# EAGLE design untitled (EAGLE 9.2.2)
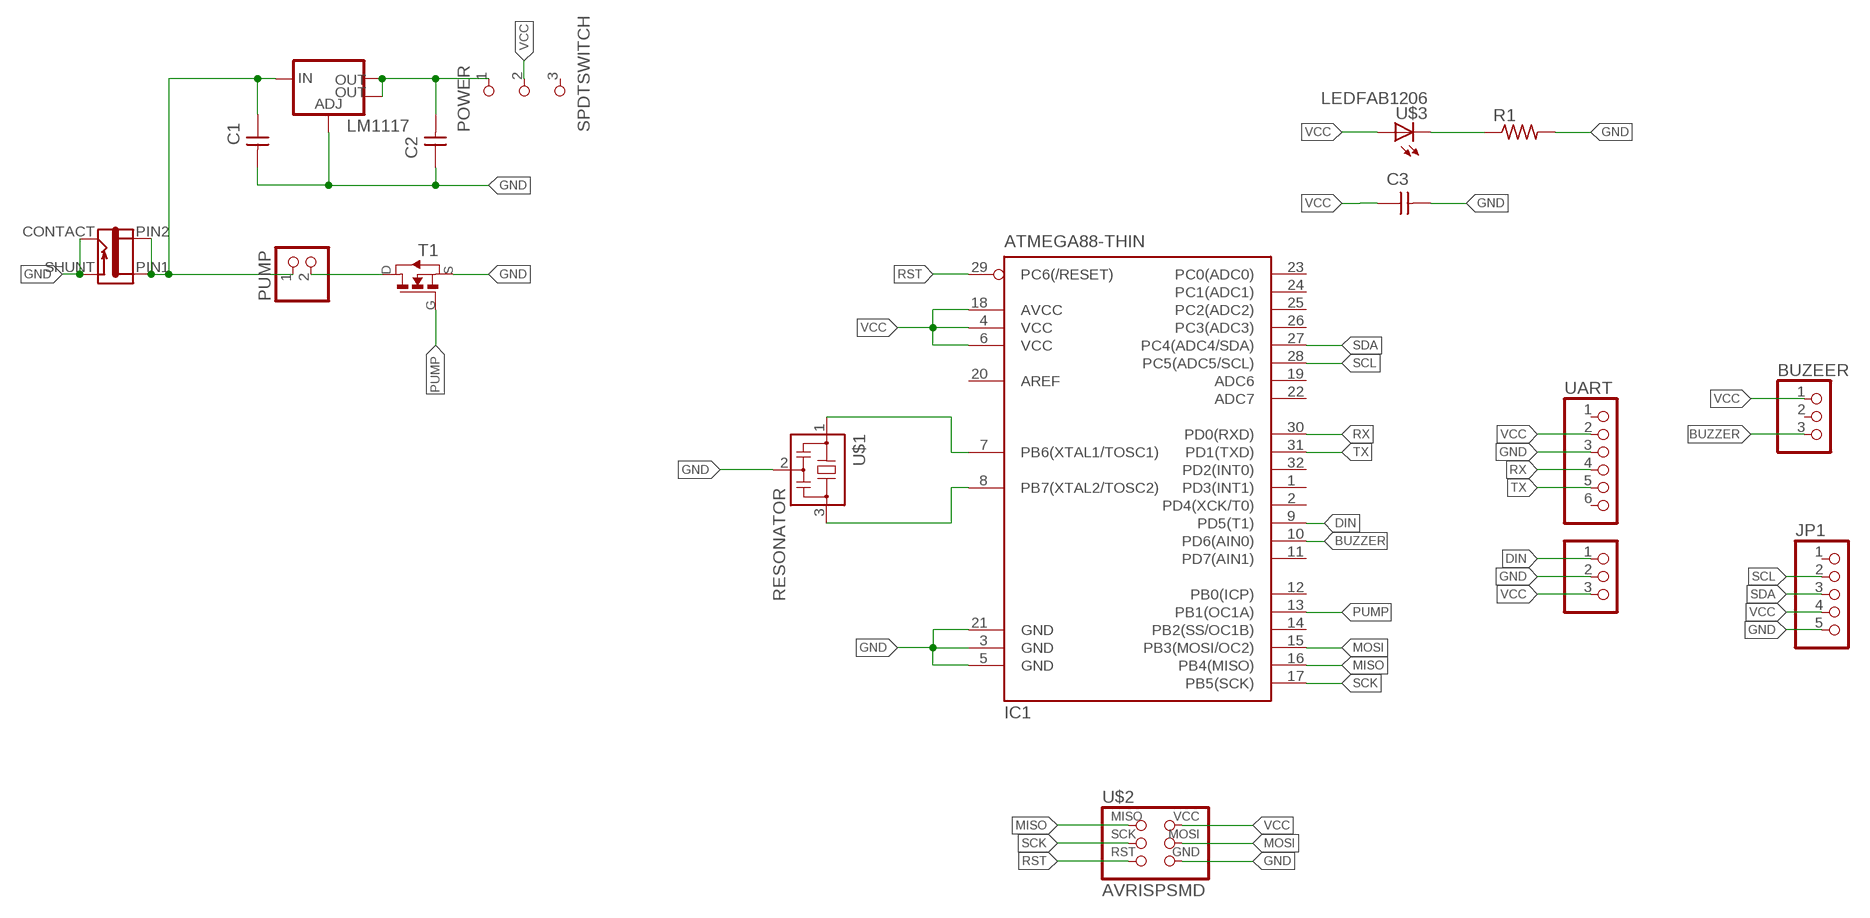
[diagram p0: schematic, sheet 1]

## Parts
BUZEER  PINHD-1X3/90  [1X03/90]
C1  CAP-UNPOLARIZEDFAB  [C1206FAB]
C2  CAP-UNPOLARIZEDFAB  [C1206FAB]
C3  CAP-UNPOLARIZEDFAB  [C1206FAB]
IC1  ATMEGA88-THIN  [TQFP32-08THIN]
J1  JACK-2.1MM  [PJ-002AH-SMT]
JP1  PINHD-1X5/90  [1X05/90]
LM1117  V_REG_LM1117SOT223  [SOT223]
NEO  PINHD-1X3/90  [1X03/90]
POWER  SPDTSWITCH  [SPDTSWITCH]
PUMP  PINHD-1X2  [1X02]
R1  RES-US1206FAB  [R1206FAB]
T1  NMOSFETTO252  [TO252]
U$1  RESONATOR  [EFOBM]
U$2  AVRISPSMD  [2X03SMD]
U$3  LEDFAB1206  [LED1206FAB]
UART  PINHD-1X6/90  [1X06/90]

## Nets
BUZZER: BUZEER.3 IC1.10(PD6(AIN0))
DIN: IC1.9(PD5(T1)) NEO.1
GND: C1.2 C2.1 C3.2 IC1.3(GND) IC1.5(GND) IC1.21(GND) J1.CONTACT J1.SHUNT JP1.5 LM1117.1(ADJ) NEO.2 R1.2 T1.2(S) U$1.2 U$2.6(GND) UART.3
MISO: IC1.16(PB4(MISO)) U$2.1(MISO)
MOSI: IC1.15(PB3(MOSI/OC2)) U$2.4(MOSI)
N$1: C2.2 LM1117.2(OUT) LM1117.4(OUT) POWER.1
N$2: PUMP.2 T1.3(D)
N$3: C1.1 J1.PIN1 J1.PIN2 LM1117.3(IN) PUMP.1
N$4: R1.1 U$3.2(C)
N$5: IC1.7(PB6(XTAL1/TOSC1)) U$1.1
N$6: IC1.8(PB7(XTAL2/TOSC2)) U$1.3
PUMP: IC1.13(PB1(OC1A)) T1.1(G)
RST: IC1.29(PC6(/RESET)) U$2.5(RST)
RX: IC1.30(PD0(RXD)) UART.4
SCK: IC1.17(PB5(SCK)) U$2.3(SCK)
SCL: IC1.28(PC5(ADC5/SCL)) JP1.2
SDA: IC1.27(PC4(ADC4/SDA)) JP1.3
TX: IC1.31(PD1(TXD)) UART.5
VCC: BUZEER.1 C3.1 IC1.4(VCC) IC1.6(VCC) IC1.18(AVCC) JP1.4 NEO.3 POWER.2 U$2.2(VCC) U$3.1(A) UART.2
Unconnected: BUZEER.2 IC1.1(PD3(INT1)) IC1.2(PD4(XCK/T0)) IC1.11(PD7(AIN1)) IC1.12(PB0(ICP)) IC1.14(PB2(SS/OC1B)) IC1.19(ADC6) IC1.20(AREF) IC1.22(ADC7) IC1.23(PC0(ADC0)) IC1.24(PC1(ADC1)) IC1.25(PC2(ADC2)) IC1.26(PC3(ADC3)) IC1.32(PD2(INT0)) JP1.1 POWER.3 UART.1 UART.6

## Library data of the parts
BUZEER NEO = pinhead:PINHD-1X3: PIN HEADER
C1-C3 = fab:CAP-UNPOLARIZED
IC1 = fab:ATMEGA88-THIN
J1 = fab:JACK-2.1MM: SMD DC power jack PJ-002AH-SMT As found in the fablab inventory. Made by Zaerc.
JP1 = pinhead:PINHD-1X5: PIN HEADER
LM1117 = fab:V_REG_LM1117: Voltage Regulator LM1117 Standard adjustable voltage regulator but in SMD form. Spark Fun Electronics SKU : COM-00595; PROD_ID: VREG-08170
POWER = fab:SPDTSWITCH
PUMP = pinhead:PINHD-1X2: PIN HEADER
R1 = fab:RES-US: Resistor (US Symbol)
T1 = fab:NMOSFET: MOS FET
U$1 = fab:RESONATOR
U$2 = fab:AVRISP
U$3 = fab:LED: LED
UART = pinhead:PINHD-1X6: PIN HEADER

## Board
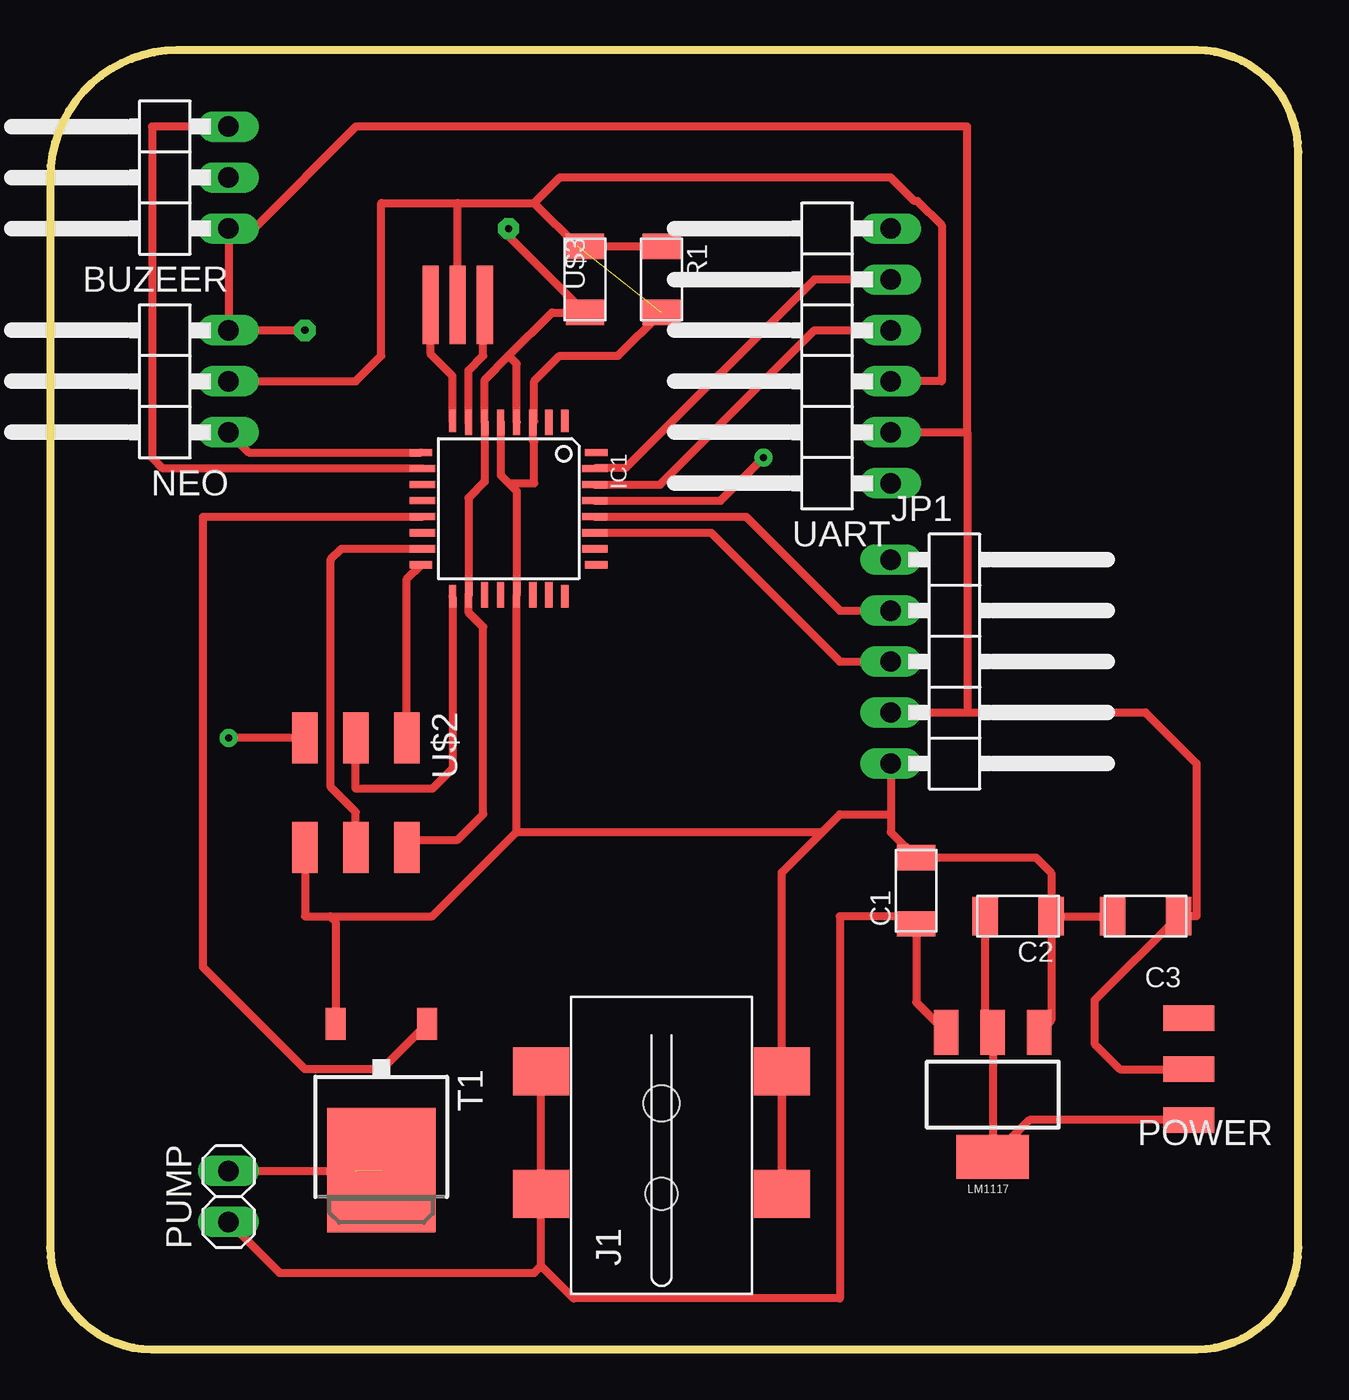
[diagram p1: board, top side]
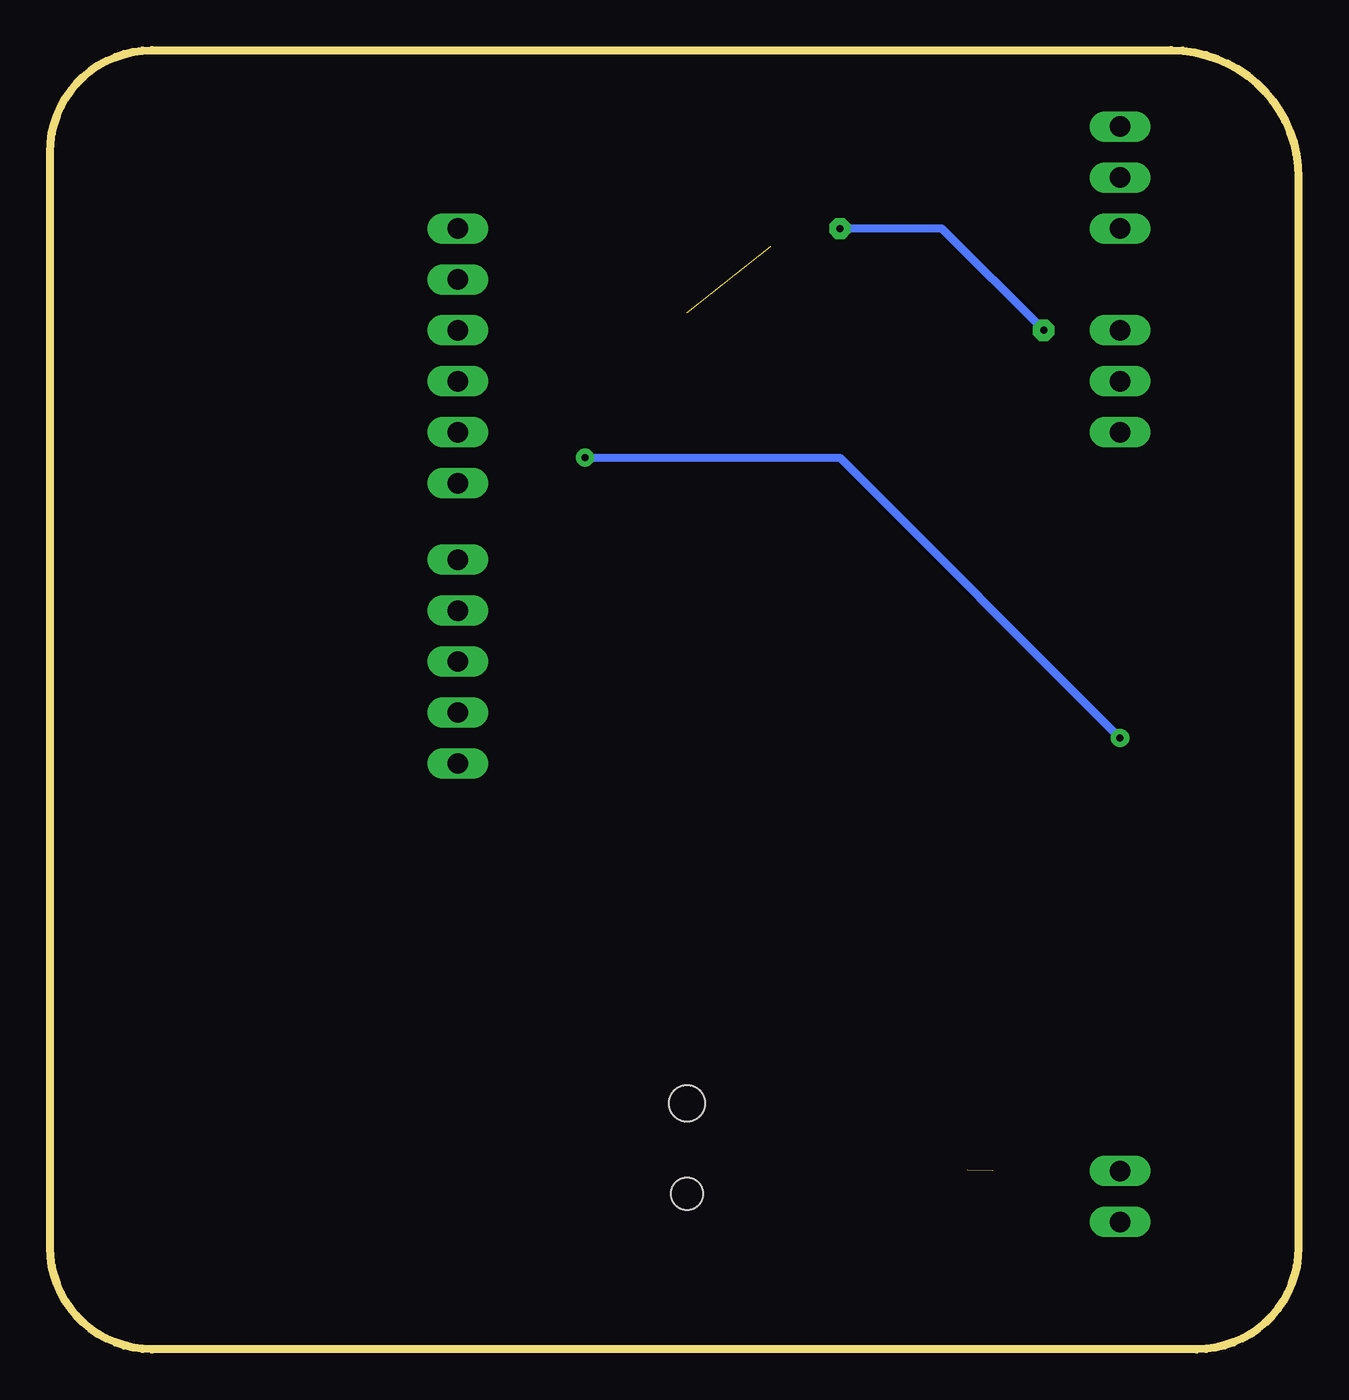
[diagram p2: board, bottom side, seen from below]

Size 62.23 x 64.77 mm. Coordinates in mm from the lower left corner, seen from the top.
Outline: 6.35,64.77 arc90 0,58.42 0,5.08 arc90 5.08,0 57.15,0 arc90 62.23,5.08 62.23,59.69 arc90 57.15,64.77 6.35,64.77
Copper layers (1*16): Top 0.035mm / dielectric 1.5mm / Bottom 0.035mm
Design rules "default *": minimum track width 16mil, minimum drill 0.35mm, track to track 16mil, track to pad 16mil, pad to pad 16mil, via to via 16mil, smd to smd 16mil, copper to edge 16mil, drill to drill 16mil, minimum pad ring 10mil, minimum via ring 8mil, stop-mask expansion 4mil, vias tented up to drill 0mil, thermal gap 10mil

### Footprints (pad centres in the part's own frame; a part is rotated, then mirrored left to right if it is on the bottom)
1X03/90 = drill 1.016 long: 1 -2.54,-3.81; 2 0,-3.81; 3 2.54,-3.81
C1206FAB = smd 1.27 x 1.905: 1 -1.651,0; 2 1.651,0
TQFP32-08THIN = smd 1.118 x 0.356: 1 -4.369,2.8; 8 -4.369,-2.8; 17 4.369,-2.8; 24 4.369,2.8 | smd 1.27 x 0.356: 2 -4.293,2; 3 -4.293,1.2; 4 -4.293,0.4; 5 -4.293,-0.4; 6 -4.293,-1.2; 7 -4.293,-2; 18 4.293,-2; 19 4.293,-1.2; 20 4.293,-0.4; 21 4.293,0.4; 22 4.293,1.2; 23 4.293,2 | smd 0.356 x 1.118: 9 -2.8,-4.369; 16 2.8,-4.369; 25 2.8,4.369; 32 -2.8,4.369 | smd 0.356 x 1.27: 10 -2,-4.293; 14 1.2,-4.293; 15 2,-4.293; 26 2,4.293; 27 1.2,4.293; 31 -2,4.293 | smd 0.35 x 1.27: 11 -1.2,-4.293; 12 -0.4,-4.293; 13 0.4,-4.293; 28 0.4,4.293; 29 -0.4,4.293; 30 -1.2,4.293
PJ-002AH-SMT = smd 2.4 x 2.8: CONTACT -2.4,-6; PIN1 3.7,6; PIN2 -2.4,6; SHUNT 3.7,-6 | hole 1.6: -2.4,0 | hole 1.8: 2.1,0
1X05/90 = drill 1.016 long: 1 -5.08,-3.81; 2 -2.54,-3.81; 3 0,-3.81; 4 2.54,-3.81; 5 5.08,-3.81
SOT223 = smd 1.219 x 2.235: 1 -2.311,-3.099; 2 0,-3.099; 3 2.311,-3.099 | smd 3.6 x 2.2: 4 0,3.099
SPDTSWITCH = smd 2.54 x 1.27: 1 0.38,2.54; 2 0.38,0; 3 0.38,-2.54
1X02 = drill 1.016 long: 1 -1.27,0; 2 1.27,0
R1206FAB = smd 1.27 x 1.905: 1 -1.651,0; 2 1.651,0
TO252 = smd 1 x 1.6: 1 -2.28,-4.8; 2 2.28,-4.8 | smd 5.4 x 6.2: 3 0,2.5
EFOBM = smd 0.8 x 3.9: 1 -1.35,0; 2 0,0; 3 1.35,0
2X03SMD = smd 2.54 x 1.27: 1 -2.54,2.54; 2 2.92,2.54; 3 -2.54,0; 4 2.92,0; 5 -2.54,-2.54; 6 2.92,-2.54
LED1206FAB = smd 1.27 x 1.905: 1 -1.651,0; 2 1.651,0
1X06/90 = drill 1.016 long: 1 -6.35,-3.81; 2 -3.81,-3.81; 3 -1.27,-3.81; 4 1.27,-3.81; 5 3.81,-3.81; 6 6.35,-3.81

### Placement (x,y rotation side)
BUZEER  5.08,58.42 90 top
C1  43.18,22.86 90 top
C2  48.26,21.59 180 top
C3  54.61,21.59 180 top
IC1  22.86,41.91 270 top
J1  30.48,10.16 90 top
JP1  45.72,34.29 270 top
LM1117  46.99,12.7 180 top
NEO  5.08,48.26 90 top
POWER  57.15,13.97 180 top
PUMP  8.89,7.62 90 top
R1  30.48,53.34 270 top
T1  16.51,11.43 180 top
U$1  20.32,52.07 180 top
U$2  15.24,27.94 270 top
U$3  26.67,53.34 90 top
UART  38.1,49.53 90 top

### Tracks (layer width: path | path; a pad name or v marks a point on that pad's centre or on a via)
BUZZER
  Top 0.406: BUZEER.3 5.08,60.96 5.08,44.45 5.62,43.91 IC1.10
DIN
  Top 0.406: NEO.1 9.9,44.71 IC1.9
GND  (1 unrouted)
  Top 0.406: U$1.2 20.32,57.15 | 20.32,57.15 24.13,57.15 | 24.13,57.15 26.29,54.99 | IC1.5 22.46,43.58 22.86,43.18 | 22.86,43.18 24.13,43.18 24.13,45.26 24.07,45.31 24.07,46.19 IC1.3 24.13,46.27 24.13,48.26 25.4,49.53 28.32,49.53 R1.2 | 24.13,57.15 25.4,58.42 41.91,58.42 43.08,57.25 43.24,57.25 44.45,56.04 44.45,48.26 UART.3 | 22.86,43.18 23.26,42.78 IC1.21 23.26,25.8 | U$2.6 12.7,21.59 13.97,21.59 | 13.97,21.59 19.05,21.59 23.26,25.8 | 13.97,21.59 14.23,21.33 T1.2 | NEO.2 15.24,48.26 16.51,49.53 16.51,57.15 20.32,57.15 | C2.1 49.91,16.41 LM1117.1 | C2.1 C3.2 | C2.1 49.91,23.75 49.15,24.51 C1.2 41.91,25.78 41.91,26.67 | JP1.5 41.91,26.67 | J1.SHUNT 36.48,8.54 35.7,7.76 | 35.56,7.62 35.7,7.76 | 35.7,7.76 J1.CONTACT 36.48,23.78 38.5,25.8 | 41.91,26.67 39.37,26.67 38.5,25.8 | 23.26,25.8 38.5,25.8
MISO
  Top 0.406: U$2.1 17.78,38.4 IC1.16
MOSI
  Top 0.406: U$2.4 15.24,26.79 13.99,28.04 13.99,39.34 13.97,39.37 14.51,39.91 IC1.15
N$1
  Top 0.406: C2.2 46.61,15.62 46.99,15.24 LM1117.2 LM1117.4 48.82,11.43 POWER.1
N$2  (1 unrouted)
  Top 0.406: PUMP.2 15.24,8.89
N$3
  Top 0.406: PUMP.1 11.43,3.81 24.13,3.81 24.48,4.16 | LM1117.3 43.18,17.3 C1.1 42.8,21.59 39.37,21.59 39.37,2.54 26.1,2.54 24.48,4.16 | 24.48,4.16 J1.PIN2 J1.PIN1
N$4
  Top 0.406: U$3.2 R1.1
N$5
  Top 0.406: U$1.1 21.59,51.99 21.59,49.53 20.86,48.8 IC1.7
N$6
  Top 0.406: 19.05,51.99 U$1.3 18.97,49.61 20.06,48.52 IC1.8
PUMP
  Top 0.406: IC1.13 7.62,41.51 7.62,19.05 12.7,13.97 16.53,13.97 T1.1
RST  (via drill 0.35 pad 0.9)
  Top 0.406: IC1.29 33.42,42.31 v35.56,44.45 | U$2.5 v8.89,30.48
  Bottom 0.406: v8.89,30.48 22.86,44.45 v35.56,44.45
RX
  Top 0.406: IC1.30 30.41,43.11 38.1,50.8 UART.4
SCK
  Top 0.406: IC1.17 20.06,28.95 19.05,27.94 15.24,27.94 U$2.3
SCL
  Top 0.406: IC1.28 34.69,41.51 39.37,36.83 JP1.2
SDA
  Top 0.406: IC1.27 32.95,40.71 39.37,34.29 JP1.3
TX
  Top 0.406: UART.5 38.1,53.34 28.68,43.92 27.16,43.92 IC1.31
VCC  (via drill 0.35 pad 1.05)
  Top 0.406: 22.86,49.53 21.66,48.33 IC1.6 21.66,43.25 20.86,42.45 IC1.18 20.87,37.61 20.87,36.73 21.59,36.01 21.59,26.67 20.32,25.4 18.16,25.4 U$2.2 | 22.86,49.53 25.02,51.69 U$3.1 22.86,55.5 v22.86,55.88 | IC1.4 23.26,49.13 22.86,49.53 | POWER.2 53.34,13.97 52.07,15.24 52.07,17.4 C3.1 57.15,21.59 57.15,29.21 54.61,31.75 45.72,31.75 | JP1.4 45.72,31.75 | UART.2 45.72,45.72 | 45.72,45.72 45.72,31.75 | 45.72,45.72 45.72,60.96 15.24,60.96 10.16,55.88 BUZEER.1 NEO.3 v12.7,50.8
  Bottom 0.406: v12.7,50.8 17.78,55.88 v22.86,55.88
